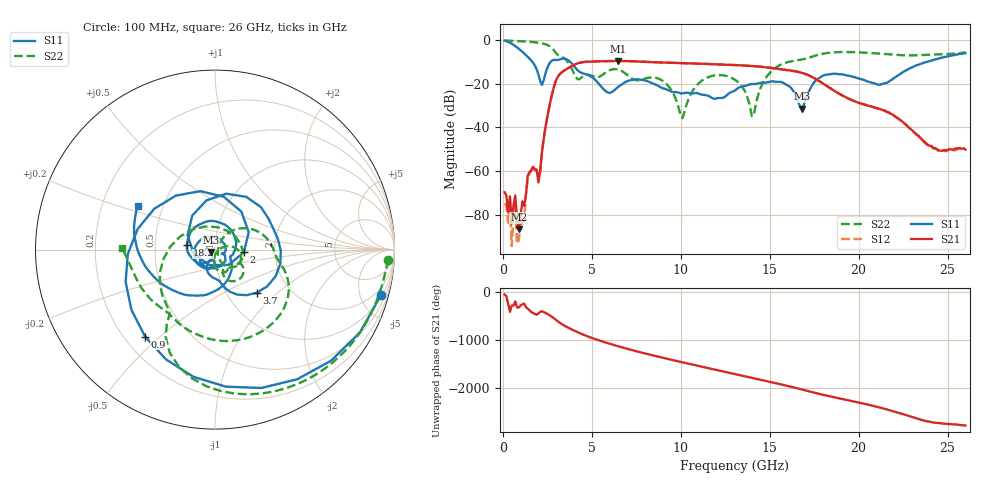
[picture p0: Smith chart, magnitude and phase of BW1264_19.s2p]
!Keysight Technologies,N5245B,MY57181159,A.13.60.06
!Date: Friday, December 18, 2020 23:52:54
!Correction: S11(Full 2 Port(1,2))
!S21(Full 2 Port(1,2))
!S12(Full 2 Port(1,2))
!S22(Full 2 Port(1,2))
!S2P File: Measurements: S11, S21, S12, S22:
# Hz S  dB  R 50
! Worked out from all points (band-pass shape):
!   260 points, 100 MHz to 26 GHz, reference 50 ohm
!   highest |S21| = -9.68 dB at 6.5 GHz (marker M1); lowest = -86.8 dB at 900 MHz (marker M2)
!   |S21| within 3 dB of the highest: 3.729 GHz to 14.89 GHz (11.16 GHz wide, 120 % of centre)
!   lowest |S11| = -31.5 dB at 16.8 GHz (marker M3), VSWR 1.05, Z = 47.7 - j1.25 ohm
!   |S11| at or under -10 dB: 1.651 GHz to 2.696 GHz (1.046 GHz wide, 48.1 % of centre); 3.772 GHz to 23.88 GHz (20.11 GHz wide, 145 % of centre)
!   |S22| runs from -35.9 to -0.3 dB; largest |S21 - S12| = 0.00066
!   S11 on the Smith chart (normalised r, x): 100 MHz: 1.15, -7.24; 900 MHz: 0.28, -0.45; 2 GHz: 1.38, -0.04; 3.7 GHz: 1.38, -0.74; 18.2 GHz: 0.73, +0.04; 26 GHz: 0.36, +0.23
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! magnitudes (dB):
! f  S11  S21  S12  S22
! 100 MHz  -0.4  -69.7  -74.9  -0.3
! 300 MHz  -1.0  -78.9  -83.7  -0.4
! 900 MHz  -4.1  -86.8  -91.4  -0.6
! 1.2 GHz  -6.3  -76.0  -83.1  -0.7
! 1.4 GHz  -7.8  -62.0  -63.7  -0.8
! 2 GHz  -15.8  -65.3  -62.6  -1.4
! 2.8 GHz  -9.3  -23.8  -23.7  -4.1
! 3.7 GHz  -9.5  -12.8  -12.8  -10.7
! 4.5 GHz  -15.4  -10.2  -10.2  -16.7
! 6.5 GHz  -21.4  -9.7  -9.7  -13.7
! 8.8 GHz  -21.4  -10.4  -10.4  -17.9
! 10.1 GHz  -24.5  -10.7  -10.7  -35.9
! 11.2 GHz  -25.1  -11.0  -11.0  -18.6
! 13.1 GHz  -22.9  -11.6  -11.6  -18.6
! 14.1 GHz  -20.2  -12.0  -12.0  -34.8
! 14.9 GHz  -19.4  -12.7  -12.7  -16.1
! 16.8 GHz  -31.5  -15.1  -15.1  -9.0
! 17.4 GHz  -20.6  -17.1  -17.1  -7.7
! 18.2 GHz  -16.0  -21.1  -21.1  -6.1
! 21.7 GHz  -19.1  -33.4  -33.2  -6.6
! 24.5 GHz  -8.6  -50.6  -51.0  -6.7
! 26 GHz  -6.1  -50.2  -49.7  -5.7
